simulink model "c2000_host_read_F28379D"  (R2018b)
settings: Solver=FixedStepDiscrete  StartTime=0.0  StopTime=inf  RelTol=1e-3  EnableMultiTasking=on
undefined symbols (not defined in the file): serial
libraries: instrumentlib x3

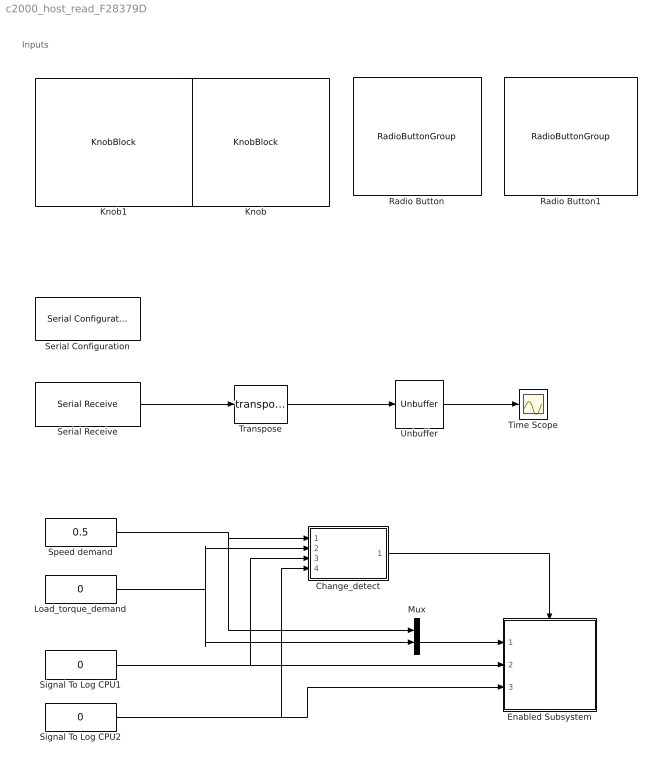
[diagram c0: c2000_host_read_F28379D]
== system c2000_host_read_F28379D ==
  note: Inputs
  Change_detect : Subsystem
  Enabled Subsystem : Subsystem  TreatAsAtomicUnit=on
  Knob : KnobBlock  WebBlockId=59  ScaleMin=-0.10000000000000001  ScaleMax=0.10000000000000001
  Knob1 : KnobBlock  WebBlockId=60  ScaleMin=0.20000000000000001  ScaleMax=0.69999999999999996
  Load_torque_demand : Constant  Value=0  VectorParams1D=off  OutDataTypeStr=fixdt(1,16,15)  SampleTime=0.03
  Mux : Mux  Inputs=2
  Radio Button : RadioButtonGroup  WebBlockId=43  SelectedLabel=Current (Ia)  ButtonGroupName=Group
  Radio Button1 : RadioButtonGroup  WebBlockId=55  SelectedLabel=Current (Ia)  ButtonGroupName=Group
  Serial Configuration : instrumentlib/Serial Configuration  Priority=-200000  ComPortMenu=COM11  ComPort=COM11  ObjConstructor=serial('COM11');  BaudRate=12000000  DataBits=8  Parity=none  StopBits=1  FlowControl=hardware  Timeout=2  ByteOrder=LittleEndian
  Serial Receive : instrumentlib/Serial Receive  ComPortMenu=COM11  ComPort=COM11  ObjConstructor=serial('COM11');  Header=SS  Terminator=EE  DataSize="[2  12000]"  DataType=uint16  EnableBlockingMode=on  ActionDataUnavailable=Output last received value  CustomValue=3  SampleTime=0.06
  Signal To Log CPU1 : Constant  Value=0  VectorParams1D=off  OutDataTypeStr=uint16  SampleTime=0.03
  Signal To Log CPU2 : Constant  Value=0  VectorParams1D=off  OutDataTypeStr=uint16  SampleTime=0.03
  Speed demand : Constant  Value=0.5  VectorParams1D=off  OutDataTypeStr=fixdt(1,16,15)  SampleTime=0.03
  Time Scope : Scope
  Transpose : Math  Operator=transpose
  Unbuffer : Unbuffer
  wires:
  Serial Receive/1 -> Transpose/1
  Unbuffer/1 -> Time Scope/1
  Transpose/1 -> Unbuffer/1
  Speed demand/1 -> Mux/1, Change_detect/1(In1)
  Load_torque_demand/1 -> Mux/2, Change_detect/2(In2)
  Change_detect/1(Out1) -> Enabled Subsystem/Enable
  Mux/1 -> Enabled Subsystem/1(In1)
  Signal To Log CPU1/1 -> Change_detect/3(In3), Enabled Subsystem/2(In2)
  Signal To Log CPU2/1 -> Change_detect/4(In4), Enabled Subsystem/3(In3)

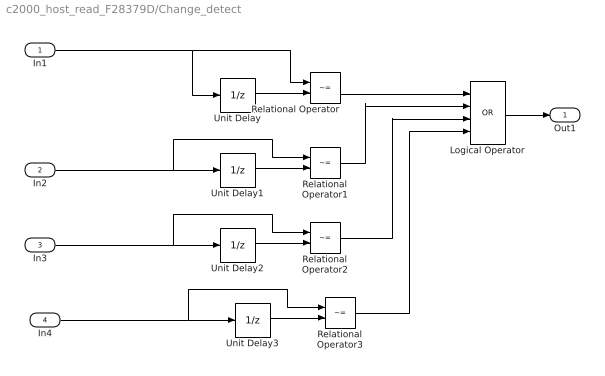
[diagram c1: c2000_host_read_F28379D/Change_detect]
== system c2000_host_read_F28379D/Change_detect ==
  In1 : Inport
  In2 : Inport  Port=2
  In3 : Inport  Port=3
  In4 : Inport  Port=4
  Logical Operator : Logic  Operator=OR  Inputs=4  AllPortsSameDT=off  OutDataTypeStr=boolean
  Relational Operator{,1..3} (4 alike) : RelationalOperator  Operator=~=  OutDataTypeStr=boolean
  Unit Delay : UnitDelay  InitialCondition=0.5  SampleTime=-1
  Unit Delay1 : UnitDelay  SampleTime=-1
  Unit Delay2 : UnitDelay  SampleTime=-1
  Unit Delay3 : UnitDelay  SampleTime=-1
  Out1 : Outport
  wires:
  In2/1 -> Relational Operator1/1, Unit Delay1/1
  Relational Operator1/1 -> Logical Operator/2
  Unit Delay1/1 -> Relational Operator1/2
  Unit Delay/1 -> Relational Operator/2
  In1/1 -> Unit Delay/1, Relational Operator/1
  Relational Operator/1 -> Logical Operator/1
  Logical Operator/1 -> Out1/1
  Unit Delay2/1 -> Relational Operator2/2
  In3/1 -> Unit Delay2/1, Relational Operator2/1
  Relational Operator2/1 -> Logical Operator/3
  In4/1 -> Relational Operator3/1, Unit Delay3/1
  Unit Delay3/1 -> Relational Operator3/2
  Relational Operator3/1 -> Logical Operator/4

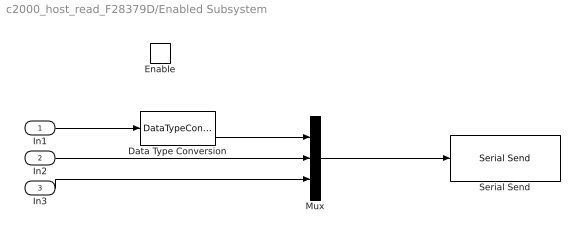
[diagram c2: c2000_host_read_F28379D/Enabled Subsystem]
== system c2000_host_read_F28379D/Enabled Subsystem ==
  In1 : Inport
  In2 : Inport  Port=2
  In3 : Inport  Port=3
  Enable : EnablePort
  Data Type Conversion : DataTypeConversion  OutDataTypeStr=uint16  ConvertRealWorld=Stored Integer (SI)
  Mux : Mux  Inputs=3
  Serial Send : instrumentlib/Serial Send  ComPortMenu=COM11  ComPort=COM11  ObjConstructor=serial('COM11');  Terminator=<none>  EnableBlockingMode=off
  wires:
  In1/1 -> Data Type Conversion/1
  Data Type Conversion/1 -> Mux/1
  In2/1 -> Mux/2
  Mux/1 -> Serial Send/1
  In3/1 -> Mux/3
